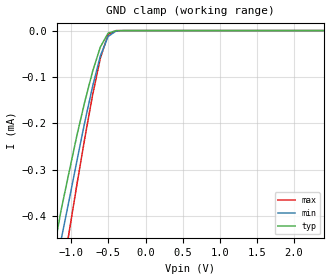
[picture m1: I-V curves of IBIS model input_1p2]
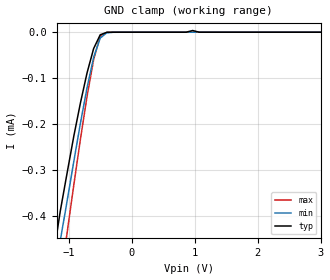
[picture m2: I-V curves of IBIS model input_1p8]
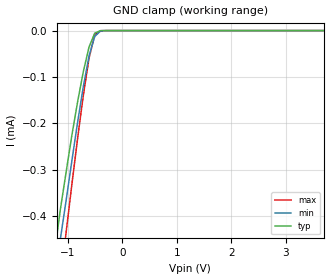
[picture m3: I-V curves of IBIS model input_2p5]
| Texas Instruments Incorporated
| SN74LXC8T245 8-Bit Dual Supply Voltage Translator
| with 3-State outputs and Schmitt-trigger Inputs
[IBIS Ver]   4.1
[File name]   sn74lxc8t245.ibs
[File Rev]   1.0
[Date]   04/24/2019
[Source]
| Texas Instruments Incorporated.
| Analog-eLab Design Center, HPA
| 12500 TI Blvd
| Dallas, TX -75243
[Notes]   Revision History:
| Rev 1.0: 09/01/2020
| - Initial version of the model
| - Model generated from simulations in SPECTRE
| - C_comp although listed in numerical order of value are
|   obtained from varying PVT conditions. For PVT conditions for
|   each specific value refer the buffer description under
|   respective [Model]. IBIS model user is responsible for using
|   appropriate C_comp to simulate for Signal Integrity.
| - Warnings regarding combined Non-monotonicity of various models have been
|   reviewd and considered minor and can be ignored.
| - Model names with a trailing _2p5 contain the model for 2.5V operation.
[Disclaimer]
| This model is designed as an aid for customers of Texas Instruments.
| TI and its licensors and suppliers make no warranties, either expressed
| or implied, with respect to this  model, including the warranties of
| merchantability or fitness for a particular purpose. The model is
| provided solely on an "as is" basis. The entire risk as to its quality
| and performance is with the customer.
| This model is subject to change without notice. Texas Instruments
| Incorporated is not responsible for updating this model.
[Copyright]
 (C) Copyright 2020 Texas Instruments Incorporated.All rights reserved.
|  Component SN74LXC8T245PW 24-Pin TSSOP - PW package
|  Part # SN74LXC8T245PWR
[Component]   SN74LXC8T245PW
[Manufacturer]   TI
[Package]   |24 TSSOP - PW package
|   typ   min   max
R_pkg   3.900e-02   3.000e-02   4.600e-02
L_pkg   2.685e-09   2.367e-09   3.177e-09
C_pkg   3.200e-13   2.520e-13   4.340e-13
[Pin]   signal_name   model_name   R_pin   L_pin   C_pin
1   VCCA   power   3.700e-02   3.153e-09   4.340e-13
2   DIR   input   3.400e-02   2.629e-09   3.410e-13
3   A1   I/O   3.200e-02   2.860e-09   3.470e-13
4   A2   I/O   4.200e-02   2.741e-09   2.900e-13
5   A3   I/O   4.600e-02   2.600e-09   2.620e-13
6   A4   I/O   4.300e-02   2.414e-09   2.660e-13
7   A5   I/O   4.200e-02   2.367e-09   2.620e-13
8   A6   I/O   4.400e-02   2.461e-09   2.520e-13
9   A7   I/O   4.200e-02   2.543e-09   2.740e-13
10   A8   I/O   3.000e-02   2.616e-09   3.320e-13
11   GND   gnd   3.700e-02   2.670e-09   3.460e-13
12   GND   gnd   3.900e-02   3.177e-09   4.330e-13
13   GND   gnd   3.700e-02   3.111e-09   4.310e-13
14   B8   I/O   3.700e-02   2.656e-09   3.450e-13
15   B7   I/O   3.100e-02   2.739e-09   3.400e-13
16   B6   I/O   4.200e-02   2.649e-09   2.820e-13
17   B5   I/O   4.600e-02   2.532e-09   2.570e-13
18   B4   I/O   4.400e-02   2.425e-09   2.660e-13
19   B3   I/O   4.400e-02   2.425e-09   2.660e-13
20   B2   I/O   4.600e-02   2.532e-09   2.570e-13
21   B1   I/O   4.200e-02   2.648e-09   2.820e-13
22   NOE   input   3.100e-02   2.738e-09   3.390e-13
23   VCCB   power   3.600e-02   2.653e-09   3.440e-13
24   VCCB   power   3.700e-02   3.110e-09   4.310e-13
|  Component SN74LXC8T245RHL 24-Pin VQFN - RHL package
|  Part # SN74LXC8T245RHLR
[Component]   SN74LXC8T245RHL
[Manufacturer]   TI
[Package]   |24 VQFN - RHL package
|   typ   min   max
R_pkg   3.700e-02   2.500e-02   5.300e-02
L_pkg   8.060e-10   5.310e-10   1.139e-09
C_pkg   1.880e-13   5.700e-14   3.100e-13
[Pin]   signal_name   model_name   R_pin   L_pin   C_pin
1   VCCA   power   4.700e-02   1.028e-09   3.100e-13
2   DIR   input   5.300e-02   1.139e-09   2.800e-13
3   A1   I/O   3.400e-02   7.350e-10   2.480e-13
4   A2   I/O   3.300e-02   7.260e-10   2.460e-13
5   A3   I/O   3.200e-02   6.830e-10   2.620e-13
6   A4   I/O   3.000e-02   6.550e-10   2.410e-13
7   A5   I/O   3.000e-02   6.580e-10   2.400e-13
8   A6   I/O   3.100e-02   6.770e-10   2.330e-13
9   A7   I/O   3.500e-02   7.590e-10   2.490e-13
10   A8   I/O   3.700e-02   7.990e-10   2.540e-13
11   GND   gnd   4.500e-02   9.840e-10   2.710e-13
12   GND   gnd   4.500e-02   9.870e-10   2.580e-13
13   GND   gnd   4.100e-02   8.860e-10   2.340e-13
14   B8   I/O   4.700e-02   1.014e-09   2.510e-13
15   B7   I/O   3.600e-02   7.740e-10   2.390e-13
16   B6   I/O   3.600e-02   7.870e-10   2.540e-13
17   B5   I/O   3.200e-02   7.070e-10   2.350e-13
18   B4   I/O   2.900e-02   6.430e-10   2.300e-13
19   B3   I/O   3.000e-02   6.450e-10   2.300e-13
20   B2   I/O   3.300e-02   7.100e-10   2.360e-13
21   B1   I/O   3.800e-02   8.150e-10   2.570e-13
22   NOE   input   3.600e-02   7.750e-10   2.390e-13
23   VCCB   power   4.700e-02   1.015e-09   2.510e-13
24   VCCB   power   4.100e-02   8.850e-10   2.360e-13
|  Component SN74LXC8T245RJW 24-Pin UQFN - RJW package
|  Part # SN74LXC8T245RJWR
[Component]   SN74LXC8T245RJW
[Manufacturer]  TI
[Package]   |24 uQFN - RJW package
|   typ   min   max
R_pkg   0.078075   0.04588   0.12141
L_pkg   0.978537917nH   0.60336nH   1.54474nH
C_pkg   0.304233333pF   0.23351pF   0.36249pF
[Pin]  signal_name model_name   R_pin   L_pin   C_pin
1   DIR   input   0.11918   1.51673nH   0.27692pF
2   A1   I/O   0.10353   1.29938nH   0.30726pF
3   A2   I/O   0.08751   1.07368nH   0.36249pF
4   A3   I/O   0.07203   0.86586nH   0.33880pF
5   A4   I/O   0.05935   0.69679nH   0.32139pF
6   A5   I/O   0.0523   0.60336nH   0.31235pF
7   A6   I/O   0.05388   0.62418nH   0.31443pF
8   A7   I/O   0.06332   0.74959nH   0.32669pF
9   A8   I/O   0.07633   0.93332nH   0.25699pF
10   GND   gnd   0.09587   1.19534nH   0.23351pF
11   GND   gnd   0.08919   1.06264nH   0.27090pF
12   GND   gnd   0.04588   0.78601nH   0.30916pF
13   B8   I/O   0.0958   1.19956nH   0.23938pF
14   B7   I/O   0.08139   1.00661nH   0.26883pF
15   B6   I/O   0.06751   0.81220nH   0.33269pF
16   B5   I/O   0.05632   0.66473nH   0.31784pF
17   B4   I/O   0.05189   0.60699nH   0.31231pF
18   B3   I/O   0.05639   0.66565nH   0.31794pF
19   B2   I/O   0.06763   0.81366nH   0.33284pF
20   B1   I/O   0.0824   1.01033nH   0.35462pF
21   NOE   input   0.09804   1.22986nH   0.28985pF
22   VCCB   power   0.12141   1.54474nH   0.26570pF
23   VCCB   power   0.1169   1.43698nH   0.29681pF
24   VCCA   power   0.05975   1.08672nH   0.34190pF
|   Model Selectors
[Model Selector] input
input_1p2   1.2V   digital input
input_1p8   1.8V   digital input
input_2p5   2.5V   digital input
input_3p3   3.3V   digital input
input_5p0   5.0V   digital input
[Model Selector] I/O
io_1p2   1.2V   Vcc
io_1p8   1.8V   Vcc
io_2p5   2.5V   Vcc
io_3p3   3.3V   Vcc
io_5p0   5.0V   Vcc
| Models and submodels in the file (10): input_1p2 (Input), input_1p8 (Input), input_2p5 (Input), input_3p3 (Input), input_5p0 (Input), io_1p2 (I/O), io_1p8 (I/O), io_2p5 (I/O), io_3p3 (I/O), io_5p0 (I/O)
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|   input_1p2 Model
[Model]   input_1p2
Model_type   Input
Vinl = 0.2
Vinh = 0.9
|   typ   min   max
C_comp   0.119pF   0.105pF   0.126pF
[Voltage Range]   1.2   1.08   1.32
|Junction Temperature
[Temperature Range]   25   125   -40
[GND Clamp Reference]   0   0   0
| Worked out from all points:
|   GND clamp passes 1 mA (typ) near -1.81 V on its own axis
[GND Clamp]
|   Voltage   I(typ)   I(min)   I(max)
-2.5V     -1.66mA    -1.64mA    -2.09mA
-1.24V    -478uA     -541uA     -650uA
-1.14V    -389uA     -453uA     -542uA
-1.03V    -305uA     -366uA     -435uA
-925mV    -226uA     -281uA     -332uA
-820mV    -154uA     -198uA     -233uA
-715mV    -88.7uA    -121uA     -140uA
-610mV    -35.6uA    -54.9uA    -59.7uA
-505mV    -5.5uA     -12.7uA    -8.49uA
-400mV    -210nA     -1.13uA    -141nA
8V        3.62nA     3.43nA     4.23nA
|   input_1p8 Model
[Model]   input_1p8
Model_type   Input
Vinl = 0.7
Vinh = 1.1
|   typ   min   max
C_comp   3.13pF   2.65pF   3.82pF
| Where Nom  PVT is Nominal Process, 2.25V, 27C
|   Fast PVT is Strong Process,  2.50V, -55C
|   Slow PVT is Weak Process,   2.0V, 150C
[Voltage Range]   1.8   1.62   1.98
|Junction Temperature
[Temperature Range]   25   125   -40
[GND Clamp Reference]   0   0   0
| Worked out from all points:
|   GND clamp passes 1 mA (typ) near -1.81 V on its own axis
[GND Clamp]
|   Voltage   I(typ)   I(min)   I(max)
-2.5V     -1.66mA    -1.64mA    -2.09mA
-1.24V    -478uA     -541uA     -650uA
-1.14V    -389uA     -453uA     -542uA
-1.03V    -305uA     -366uA     -435uA
-820mV    -154uA     -198uA     -233uA
-715mV    -88.7uA    -121uA     -140uA
-610mV    -35.6uA    -54.9uA    -59.7uA
-505mV    -5.5uA     -12.7uA    -8.49uA
-400mV    -210nA     -1.13uA    -141nA
965mV     3.74uA     3.02nA     4.93nA
1.07V     3.25nA     2.95nA     3.92nA
8V        3.62nA     3.43nA     4.23nA
|   input_2p5 Model
[Model]   input_2p5
Model_type   Input
Vinl = 1.0
Vinh = 1.4
|   typ   min   max
C_comp   3.03pF   2.54pF   3.83pF
| Where Nom  PVT is Nominal Process, 2.25V, 27C
|   Fast PVT is Strong Process,  2.50V, -55C
|   Slow PVT is Weak Process,   2.0V, 150C
[Voltage Range]   2.5   2.25   2.75
|Junction Temperature
[Temperature Range]   25   125   -40
[GND Clamp Reference]   0   0   0
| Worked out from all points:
|   GND clamp passes 1 mA (typ) near -1.81 V on its own axis
[GND Clamp]
|   Voltage   I(typ)   I(min)   I(max)
-2.5V     -1.66mA    -1.64mA    -2.09mA
-1.24V    -478uA     -541uA     -650uA
-1.14V    -389uA     -453uA     -542uA
-1.03V    -305uA     -366uA     -435uA
-925mV    -226uA     -281uA     -332uA
-820mV    -154uA     -198uA     -233uA
-715mV    -88.7uA    -121uA     -140uA
-610mV    -35.6uA    -54.9uA    -59.7uA
-505mV    -5.5uA     -12.7uA    -8.49uA
-400mV    -210nA     -1.14uA    -141nA
8V        3.62nA     3.43nA     4.23nA
